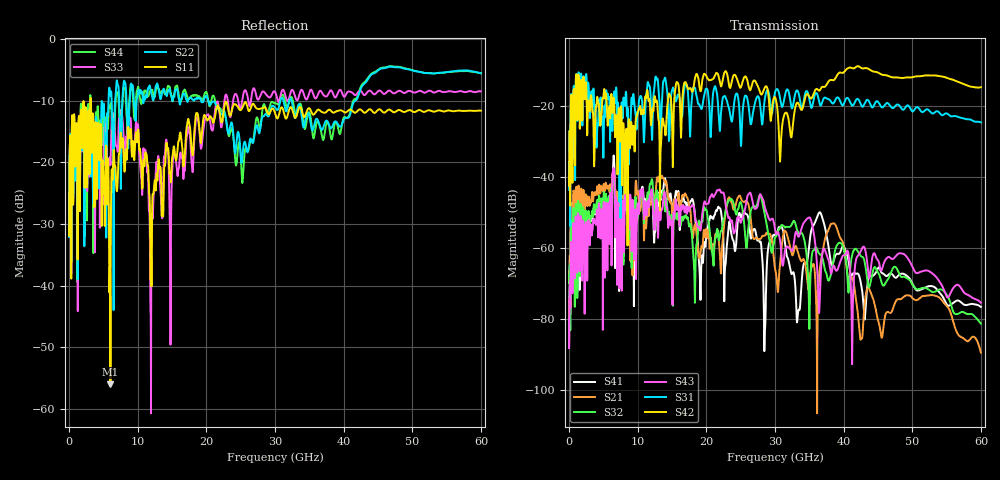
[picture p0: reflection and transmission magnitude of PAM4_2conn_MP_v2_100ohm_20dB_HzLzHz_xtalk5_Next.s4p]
! Info: Touchstone file created by Circ.  Input file=FAB50GbE_2conn_Midplane_Examax_Topo2_v2_100ohm_20dB_HzLzHz.circ
# Hz S RI R 50
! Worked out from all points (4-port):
!   6000 points, 10 MHz to 60 GHz, reference 50 ohm
!   strongest paths, dB at 10 MHz, 15.01 GHz, 30.01 GHz, 45.01 GHz, 60 GHz:
!     S42: -42.5, -25.2, -17.5, -10.5, -14.7
!     S31: -43.6, -15.5, -16.1, -18.8, -24.6
!     S43: -88.3, -56.8, -54.8, -63.5, -75.5
!     S32: -70.0, -54.0, -57.2, -66.9, -81.4
!     S21: -69.6, -49.7, -65.9, -80.4, -89.6
!     S41: -88.2, -48.4, -56.5, -65.8, -76.7
!   lowest |S11| = -56.0 dB at 6.03 GHz (marker M1), VSWR 1.00, Z = 50.1 - j0.13 ohm
!   |S11| at or under -10 dB: start of sweep to 3.111 GHz; 3.183 GHz to end of sweep
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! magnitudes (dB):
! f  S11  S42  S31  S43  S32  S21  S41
! 10 MHz  -31.9  -42.5  -43.6  -88.3  -70.0  -69.6  -88.2
! 1.23 GHz  -26.5  -21.0  -23.5  -56.7  -55.6  -52.0  -53.2
! 6.03 GHz  -56.0  -22.0  -24.4  -44.5  -45.0  -42.2  -45.2
! 11.94 GHz  -35.0  -25.4  -20.7  -44.3  -41.8  -47.2  -46.0
! 18.28 GHz  -14.7  -12.8  -14.8  -50.3  -69.5  -53.7  -49.5
! 22.86 GHz  -10.2  -10.2  -17.9  -48.5  -48.7  -49.7  -63.2
! 60 GHz  -11.6  -14.7  -24.6  -75.5  -81.4  -89.6  -76.7
